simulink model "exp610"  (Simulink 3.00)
settings: Solver=ode45  StartTime=0.0  StopTime=10.0  RelTol=1e-3
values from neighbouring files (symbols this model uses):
  A = [0 1 0;0 -1.799 6.953;0 0.939 -1.660]    [EXP6_10.M]    (also in EXP6_8.M = [a11 a12 0 -g;a21 a22 1 0;a31 a31 a33 0;0 1 0 0]; EXP6_9.m = [a11 a12 0 -g;a21 a22 1 0;a31 a31 a33 0;0 1 0 0]; EXP7_1.M = [0 1 0 0;0 0 -mb*g/(1-mb) 0;0 0 0 1;0 0 m2_bar*g/(1-mb) 0]; EXP7_2.M = [0 1 0 0;0 0 -mb*g/(1-mb) 0;0 0 0 1;0 0 m2_bar*g/(1-mb) 0])
  B = [0 0;-28.97 -6.453;-0.174 -0.230]    [EXP6_10.M]    (also in EXP6_8.M = [b1;b2;b3;0]; EXP6_9.m = [b1;b2;b3;0]; EXP7_1.M = [0;1/((m+M)*(1-mb));0;-m2_bar/((m+M)*(1-mb))]; EXP7_2.M = [0;1/((m+M)*(1-mb));0;-m2_bar/((m+M)*(1-mb))])
  K = Q*inv(V)    [EXP6_10.M]    (also in EXP6_8.M = acker(A,B,P); EXP6_9.m = acker(A_bar,B_bar,P); EXP7_3.M = acker(A,B,Pc); Exp7_4.m = [0.922 -6.5955 -2.35 -8.977])
libraries: simulink3 x3

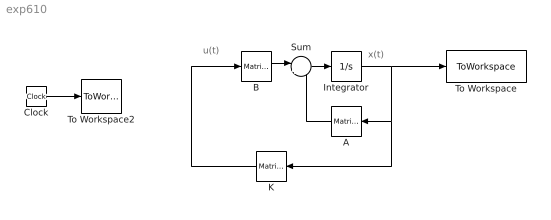
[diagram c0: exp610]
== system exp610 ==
  note: x(t)
  note: u(t)
  A : simulink3/Math/Matrix Gain  Orientation=left  K=A
  B : simulink3/Math/Matrix Gain  K=B
  Clock : Clock
  Integrator : Integrator  ExternalReset=none  InitialConditionSource=internal  InitialCondition=[0.2 .1 -0.5]  LimitOutput=off  UpperSaturationLimit=inf  LowerSaturationLimit=-inf  ShowSaturationPort=off  ShowStatePort=off  AbsoluteTolerance=auto
  K : simulink3/Math/Matrix Gain  Orientation=left  K=K
  Sum : Sum  Inputs=|++  SaturateOnIntegerOverflow=on
  To Workspace : ToWorkspace  VariableName=states  SampleTime=-1  SaveFormat=Matrix
  To Workspace2 : ToWorkspace  VariableName=time  SampleTime=-1  SaveFormat=Matrix
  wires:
  B/1 -> Sum/1
  Sum/1 -> Integrator/1
  Integrator/1 -> To Workspace/1, A/1, K/1
  A/1 -> Sum/2
  K/1 -> B/1
  Clock/1 -> To Workspace2/1
